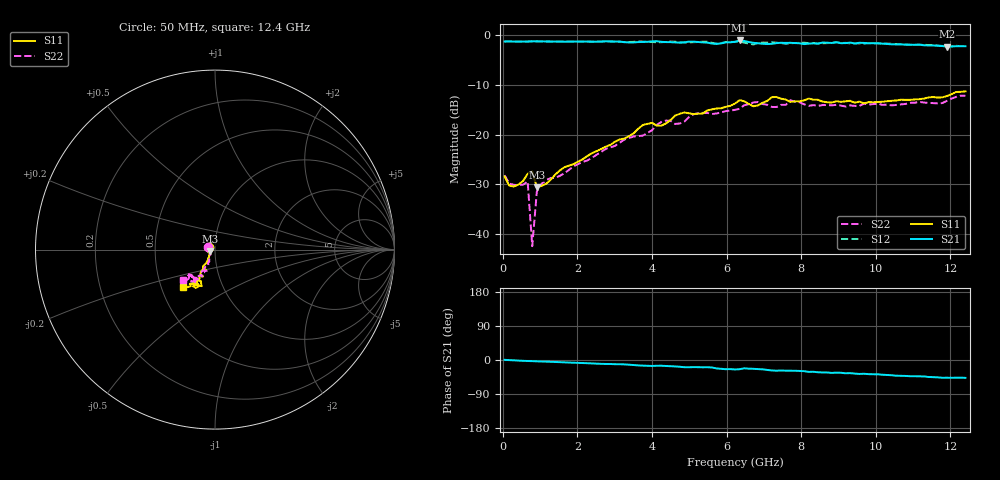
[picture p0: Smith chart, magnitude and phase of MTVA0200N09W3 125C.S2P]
! Network Analyzer HP8720D.06.14 Serial No. US36140669
! 24 Jul 2008  11:27:00
! Frequency  S11  S21  S12  S22
# HZ  S  DB R 50
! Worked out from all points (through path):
!   101 points, 50 MHz to 12.4 GHz, reference 50 ohm
!   highest |S21| = -1.05 dB at 6.348 GHz (marker M1); lowest = -2.3 dB at 11.91 GHz (marker M2)
!   group delay of S21, straight-line fit = 10.8 ps
!   lowest |S11| = -30.6 dB at 914.5 MHz (marker M3), VSWR 1.06, Z = 47.3 - j0.957 ohm
!   |S11| at or under -10 dB: start of sweep to end of sweep
!   |S22| runs from -42.4 to -12.2 dB; largest |S21 - S12| = 0.047
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5e7  -28.41 157.4  -1.26 0.4  -1.27 0.2  -28.16 158.1
2.97e8  -30.46 -178.3  -1.27 -0.8  -1.28 -1.0  -30.09 -179.2
6.675e8  -27.87 -158.5  -1.28 -2.6  -1.25 -2.6  -29.44 -177.0
7.91e8  -27.41 179.3  -1.23 -3.0  -1.21 -2.8  -42.45 149.0
9.145e8  -30.60 -160.0  -1.23 -3.6  -1.25 -3.4  -31.41 -149.5
1.1615e9  -29.89 -147.9  -1.25 -4.3  -1.28 -4.4  -29.15 -143.3
1.6555e9  -26.55 -134.6  -1.29 -6.2  -1.26 -6.2  -27.76 -130.4
2.1495e9  -24.93 -128.6  -1.28 -8.1  -1.26 -8.1  -25.49 -121.9
3.261e9  -20.79 -122.6  -1.39 -11.6  -1.39 -12.2  -20.98 -115.4
3.755e9  -18.07 -121.7  -1.35 -14.8  -1.26 -13.6  -20.20 -115.4
4.249e9  -18.21 -118.9  -1.32 -15.1  -1.41 -16.3  -17.47 -115.4
4.8665e9  -15.54 -116.0  -1.42 -19.1  -1.50 -18.0  -17.39 -120.1
5.237e9  -15.80 -116.2  -1.35 -18.9  -1.37 -20.0  -15.68 -118.1
6.225e9  -13.75 -119.7  -1.31 -25.0  -1.35 -23.3  -15.02 -123.0
6.3485e9  -13.06 -117.3  -1.05 -24.3  -1.23 -22.9  -14.80 -125.5
6.719e9  -14.30 -113.8  -1.53 -23.2  -1.87 -25.0  -13.53 -124.1
7.213e9  -12.46 -120.9  -1.72 -27.6  -1.38 -26.6  -14.43 -120.4
7.707e9  -13.41 -116.2  -1.52 -28.3  -1.64 -29.5  -13.08 -127.0
8.3245e9  -12.97 -119.0  -1.64 -31.0  -1.56 -30.6  -14.06 -126.5
1.0424e10  -13.20 -122.9  -1.83 -40.2  -1.71 -40.6  -14.12 -135.4
1.1906e10  -12.23 -123.7  -2.27 -46.8  -2.26 -46.6  -13.20 -132.2
1.24e10  -11.30 -130.7  -2.21 -47.1  -2.14 -47.0  -12.19 -136.2
